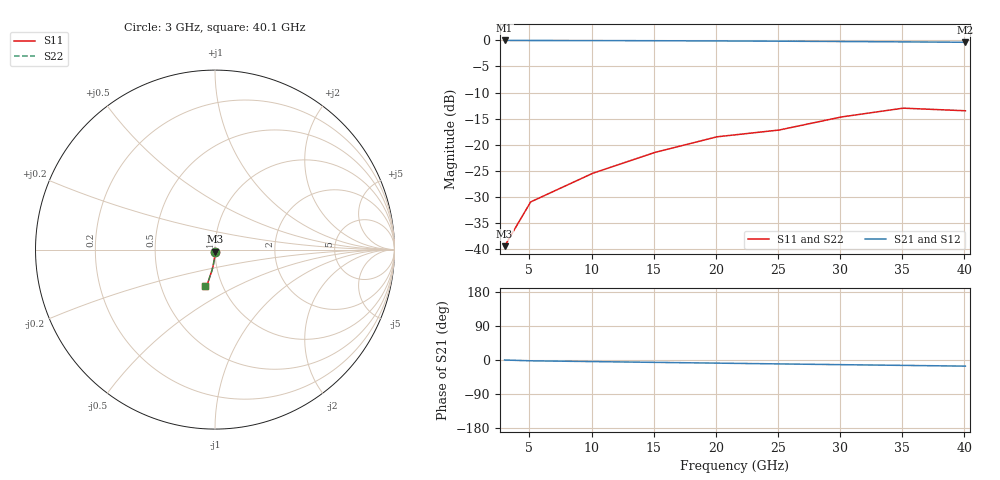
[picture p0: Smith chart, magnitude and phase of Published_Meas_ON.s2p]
! Created Wed May 09 09:19:32 2001
# hz S db R 50
! SP2.SP
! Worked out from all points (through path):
!   9 points, 3 GHz to 40.1 GHz, reference 50 ohm
!   highest |S21| = 0.00 dB at 3 GHz (marker M1); lowest = -0.4 dB at 40.1 GHz (marker M2)
!   lowest |S11| = -39.5 dB at 3 GHz (marker M3), VSWR 1.02, Z = 50 - j1.06 ohm
!   |S11| at or under -10 dB: start of sweep to end of sweep
!   |S22| runs from -39.5 to -13.0 dB; largest |S21 - S12| = 0
3e9  -39.50 -90.0  -0.00 -0.0  -0.00 -0.0  -39.50 -90.0
5.1e9  -31.00 -92.1  -0.01 -2.1  -0.01 -2.1  -31.00 -92.1
1.01e10  -25.50 -94.2  -0.02 -4.2  -0.02 -4.2  -25.50 -94.2
1.51e10  -21.50 -96.2  -0.05 -6.2  -0.05 -6.2  -21.50 -96.2
2.01e10  -18.50 -98.3  -0.09 -8.3  -0.09 -8.3  -18.50 -98.3
2.51e10  -17.20 -100.0  -0.14 -10.3  -0.14 -10.3  -17.20 -100.0
3.01e10  -14.70 -102.0  -0.20 -12.3  -0.20 -12.3  -14.70 -102.0
3.51e10  -13.00 -104.0  -0.27 -14.2  -0.27 -14.2  -13.00 -104.0
4.01e10  -13.50 -106.0  -0.35 -16.2  -0.35 -16.2  -13.50 -106.0
